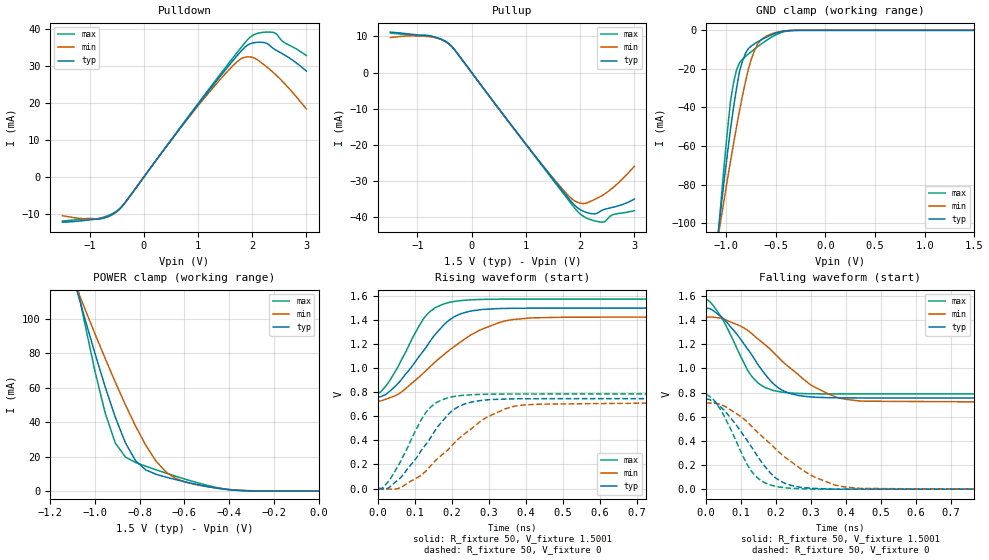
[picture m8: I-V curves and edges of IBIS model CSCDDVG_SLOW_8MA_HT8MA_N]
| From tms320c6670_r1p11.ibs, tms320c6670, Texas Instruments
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|   Model Cell CSCDDVG_SLOW_8MA_HT8MA_N
|SLOW_8MA
[Model]   CSCDDVG_SLOW_8MA_HT8MA_N
Model_type   I/O
Polarity   Non-Inverting
Enable   Active-Low
Cref =  4.0000pF
Rref =  100.0000M
Vref =  0V
Vmeas =  0.75
C_comp   1.5249p   1.4275p   1.6205p
|[mode_tieoffpin] SR0=0  SR1=1 I0=0 I1=0 I2=1
[Model Spec]
Vinl   0.6125   0.6125   0.6125
Vinh   0.9625   0.9625   0.9625
D_overshoot_high 1.95 1.95 1.95
D_overshoot_low -0.3 -0.3 -0.3
D_overshoot_time 1E-9 1E-9 1E-9
S_overshoot_high 1.575 1.575 1.575
S_overshoot_low 0 0 0
[Receiver Thresholds]
Vcross_low = 0.5625V
Vcross_high = 0.9375V
Vdiff_ac = +350mV
Vdiff_dc = +200mV
Tdiffslew_ac = 350ps
[Add Submodel]|Submodel_name Mode
DIFF_HT_TH_8MA Non-Driving
[Temperature Range]   25   105   -40
[Voltage Range]   1.5   1.425   1.575
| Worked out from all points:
|   slope of the pulldown table from 0 to 0.225 V, typ, clamps not added: 50.1 ohm
|   slope of the pullup table from 0 to 0.225 V, typ, clamps not added: 50.1 ohm
|   GND clamp passes 1 mA (typ) near -0.47 V on its own axis
|   POWER clamp passes 1 mA (typ) near -0.42 V on its own axis
|   rising waveform, R_fixture 50, V_fixture 1.5001: 20-80 % time 112ps typ, 168ps min, 83.3ps max; typ from 0.756 V to 1.5 V
|   rising waveform, R_fixture 50, V_fixture 0: 20-80 % time 108ps typ, 154ps min, 80.3ps max; typ from 0 V to 0.747 V
|   falling waveform, R_fixture 50, V_fixture 1.5001: 20-80 % time 114ps typ, 168ps min, 82.8ps max; typ from 1.5 V to 0.755 V
|   falling waveform, R_fixture 50, V_fixture 0: 20-80 % time 111ps typ, 172ps min, 80.3ps max; typ from 0.746 V to 0 V
[POWER_clamp]
|   voltage   I(typ)   I(min)   I(max)
-1.5V     321.7mA    260.6mA    415.9mA
-1.076V   114.2mA    115.8mA    116.9mA
-1.061V   107.2mA    110.9mA    107.1mA
-954.6mV  60.59mA    77.06mA    45.35mA
-909.2mV  42.85mA    63.21mA    27.81mA
-863.7mV  27.9mA     49.99mA    19.69mA
-818.2mV  17.49mA    37.63mA    16.52mA
-772.8mV  12.19mA    26.53mA    14.33mA
-681.9mV  7.985mA    10.89mA    10.33mA
-590.9mV  5.094mA    4.955mA    6.6mA
-363.7mV  298.5uA    465.2uA    297.6uA
0V        1.518nA    24.08nA    367.8pA
[Pulldown]
|   voltage   I(typ)   I(min)   I(max)
-1.5V     -12.15mA   -10.4mA    -11.83mA
-863.7mV  -11.34mA   -11.22mA   -11.25mA
-500mV    -9.267mA   -9.352mA   -9.148mA
-318.2mV  -6.354mA   -6.371mA   -6.385mA
1.046V    20.42mA    20.05mA    20.72mA
1.591V    30.47mA    29.26mA    31.18mA
1.818V    34.39mA    32.13mA    35.4mA
1.955V    35.92mA    32.45mA    37.67mA
2.091V    36.38mA    31.76mA    38.77mA
2.273V    36.08mA    29.69mA    39.15mA
2.364V    35.03mA    28.59mA    39.11mA
3V        28.64mA    18.41mA    32.82mA
[Pullup]
|   voltage   I(typ)   I(min)   I(max)
-1.5V     11.21mA    9.69mA     10.94mA
-818.2mV  10.23mA    9.978mA    10.29mA
-590.9mV  9.401mA    9.328mA    9.374mA
-409.1mV  7.828mA    7.781mA    7.859mA
1.227V    -24.14mA   -24.11mA   -24.35mA
1.727V    -33.63mA   -33.09mA   -34.13mA
1.909V    -36.81mA   -35.55mA   -37.6mA
2.046V    -38.25mA   -36.2mA    -39.57mA
2.227V    -39.04mA   -35.36mA   -40.83mA
2.409V    -38.05mA   -33.98mA   -41.36mA
2.591V    -37.29mA   -32.03mA   -39.38mA
3V        -34.98mA   -25.95mA   -38.2mA
[GND_clamp]
|   voltage   I(typ)   I(min)   I(max)
-1.5V     -310.1mA   -250.5mA   -402.5mA
-1.076V   -103.6mA   -106.2mA   -105.2mA
-1.046V   -89.81mA   -96.36mA   -86.02mA
-954.6mV  -51.22mA   -67.87mA   -36.88mA
-924.3mV  -40.08mA   -58.86mA   -27.29mA
-863.7mV  -21.24mA   -41.56mA   -16.73mA
-833.4mV  -15.8mA    -33.75mA   -15.03mA
-772.8mV  -9.345mA   -19.75mA   -12.19mA
-712.2mV  -6.928mA   -10.35mA   -9.704mA
-621.3mV  -4.261mA   -3.896mA   -6.225mA
-409.1mV  -337.1uA   -289.1uA   -618.9uA
1.5V      1.518nA    257.2nA    299pA
[Ramp]
| variable   typ   min   max
dV/dt_f   0.596016/0.16747067n   0.56408/0.25220681n   0.629272/0.12664996n
dV/dt_r 0.60150488/0.15902866n  0.5749704/0.2367164n  0.6310776/0.12226898n
R_load = 50
[Rising Waveform]
R_fixture = 50
V_fixture = 1.5001
V_fixture_min = 1.425
V_fixture_max = 1.575
|   time   V(typ)   V(min)   V(max)
0s        755.9mV    721.1mV    789.3mV
26.08ps   794.8mV    748.7mV    873mV
52.37ps   869.7mV    781.6mV    1.005V
123.7ps   1.149V     963.5mV    1.415V
154.8ps   1.283V     1.054V     1.503V
194.8ps   1.406V     1.156V     1.549V
286.6ps   1.49V      1.331V     1.572V
341.3ps   1.497V     1.392V     1.574V
405.7ps   1.499V     1.417V     1.575V
1.291ns   1.5V       1.425V     1.575V
[Rising Waveform]
R_fixture = 50
V_fixture = 0
V_fixture_min = 0
V_fixture_max = 0
|   time   V(typ)   V(min)   V(max)
0s        0V         0V         0V
16.45ps   -3.235mV   -2.5mV     18.64mV
58.93ps   85.17mV    6.841mV    215.7mV
127.9ps   362.9mV    141.9mV    628.2mV
160ps     509.3mV    246.9mV    718.7mV
198.5ps   641.5mV    354.1mV    761.4mV
231.4ps   700.1mV    449.2mV    775.4mV
291.7ps   736.3mV    588.2mV    783.7mV
389.1ps   746mV      693.6mV    785.9mV
1.298ns   747.3mV    712.8mV    786.3mV
[Falling Waveform]
R_fixture = 50
V_fixture = 1.5001
V_fixture_min = 1.425
V_fixture_max = 1.575
|   time   V(typ)   V(min)   V(max)
0s        1.499V     1.424V     1.575V
20.45ps   1.478V     1.425V     1.521V
48.81ps   1.414V     1.409V     1.398V
128.4ps   1.121V     1.293V     942.3mV
157.5ps   993.7mV    1.221V     860.6mV
197.2ps   860.3mV    1.119V     814.1mV
240.3ps   792.2mV    1.004V     796.4mV
294.3ps   764.9mV    873mV      790.6mV
395.9ps   756mV      745.7mV    788.8mV
1.291ns   755.2mV    720.6mV    788.5mV
[Falling Waveform]
R_fixture = 50
V_fixture = 0
V_fixture_min = 0
V_fixture_max = 0
|   time   V(typ)   V(min)   V(max)
0s        746.4mV    711.9mV    785.4mV
17.52ps   731.2mV    713.4mV    751.9mV
42.22ps   680.3mV    700.5mV    654.1mV
128.7ps   354.6mV    524.3mV    152.3mV
152.6ps   248.2mV    455.5mV    80.57mV
192.1ps   110.3mV    351.7mV    27.93mV
234.9ps   38.42mV    244.6mV    8.931mV
299.2ps   8.068mV    115.5mV    320.3uV
399ps     0V         17.19mV    0V
1.298ns   0V         0V         0V
